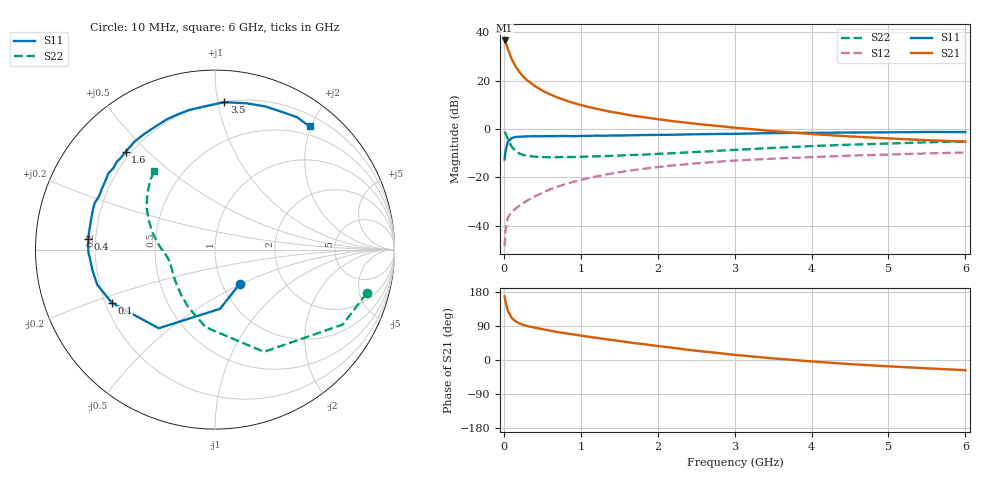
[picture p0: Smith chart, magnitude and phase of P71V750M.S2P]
! SIEMENS Small Signal Semiconductors
! BFP196
! Si NPN RF Bipolar Junction Transistor in SOT143
! VCE = 1.75 V  IC = 50 mA
! Common Emitter S-Parameters:  May  1996
# GHz  S  MA  R  50
!  f  S11  S21  S12  S22
! GHz  MAG  ANG  MAG  ANG  MAG  ANG  MAG  ANG
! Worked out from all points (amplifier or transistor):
!   36 points, 10 MHz to 6 GHz, reference 50 ohm
!   highest |S21| = 36.6 dB at 10 MHz (marker M1)
!   |S21| within 3 dB of that: start of sweep to 47.14 MHz
!   unconditionally stable (mu >= 1): 413.4 MHz to 5.023 GHz
!   at 250 MHz: K = 0.87, MSG = 26.2 dB, |S12| = -30.7 dB
!   at 1.4 GHz: K = 1.09, MAG = 10.9 dB, |S12| = -18.4 dB
!   at 6 GHz: K = 0.99, MSG = 2.2 dB, |S12| = -9.7 dB
!   S11 on the Smith chart (normalised r, x): 10 MHz: 1.21, -0.49; 100 MHz: 0.23, -0.23; 400 MHz: 0.17, +0.04; 1.6 GHz: 0.18, +0.43; 3.5 GHz: 0.20, +1.04; 6 GHz: 0.36, +1.97
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0.01  0.2353 -54.0  67.44 167.7  0.0038 79.3  0.8795 -16.0
0.02  0.3312 -85.2  62.67 155.2  0.0075 71.4  0.8252 -30.4
0.05  0.5389 -125.6  46.4 131.0  0.0147 54.6  0.6318 -64.4
0.1  0.6467 -152.7  28.47 111.6  0.0192 48.0  0.4355 -96.9
0.15  0.6847 -163.4  19.93 102.4  0.0225 48.9  0.3525 -115.2
0.2  0.693 -170.6  15.26 96.7  0.0258 51.3  0.3133 -127.3
0.25  0.6977 -175.6  12.23 92.8  0.0293 54.7  0.2915 -136.4
0.3  0.7057 -178.9  10.26 90.0  0.033 57.3  0.281 -142.2
0.4  0.7095 175.2  7.759 85.4  0.0403 60.1  0.2686 -151.1
0.5  0.7082 170.6  6.211 81.4  0.048 61.8  0.263 -156.8
0.6  0.7107 166.2  5.188 77.4  0.0567 62.6  0.2618 -160.6
0.7  0.7153 161.9  4.459 73.7  0.0645 62.9  0.2626 -163.5
0.9  0.7115 155.1  3.474 67.6  0.0809 61.8  0.2638 -168.0
1.1  0.7205 148.0  2.856 61.4  0.0968 60.2  0.2698 -171.1
1.3  0.7255 141.4  2.426 55.6  0.1127 57.7  0.2752 -174.0
1.6  0.7385 132.4  1.974 47.3  0.1354 53.7  0.2878 -177.7
2.2  0.7618 115.7  1.45 32.1  0.1769 44.9  0.3163 174.6
2.8  0.7911 100.4  1.147 18.1  0.212 36.0  0.3568 165.5
3.5  0.8231 86.4  0.905 4.3  0.2442 26.1  0.4071 155.5
4.5  0.8458 70.5  0.702 -10.9  0.2813 14.1  0.4744 143.0
5.5  0.868 58.2  0.587 -22.0  0.3136 3.2  0.5299 132.6
6  0.865 52.5  0.549 -26.8  0.3281 -2.4  0.5554 127.5
